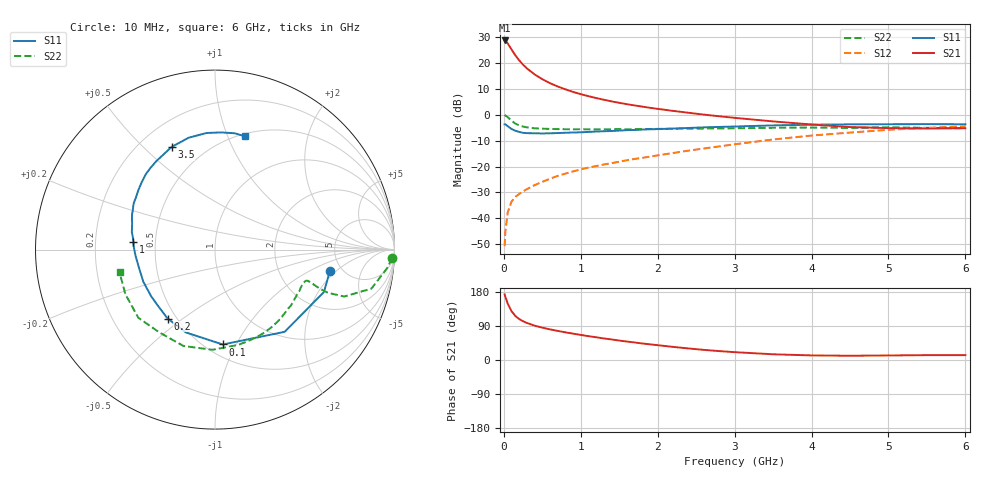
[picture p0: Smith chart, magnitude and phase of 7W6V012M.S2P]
! Infineon Technologies  Discrete & RF Semiconductors
! BFS17W
! Si NPN RF Bipolar Junction Transistor in SOT323
! VCE = 6 V  IC = 12 mA
! Common Emitter S-Parameters:  August  1999
# GHz  S  MA  R  50
!  f  S11  S21  S12  S22
! GHz  MAG  ANG  MAG  ANG  MAG  ANG  MAG  ANG
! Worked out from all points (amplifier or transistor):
!   36 points, 10 MHz to 6 GHz, reference 50 ohm
!   highest |S21| = 28.7 dB at 10 MHz (marker M1)
!   |S21| within 3 dB of that: start of sweep to 89.78 MHz
!   unconditionally stable (mu >= 1): 386.1 MHz to 2.223 GHz; 5.303 GHz to end of sweep
!   at 250 MHz: K = 0.83, MSG = 24.4 dB, |S12| = -29.6 dB
!   at 1.4 GHz: K = 1.18, MAG = 9.4 dB, |S12| = -18.7 dB
!   at 6 GHz: K = 1.04, MAG = -1.7 dB, |S12| = -4.5 dB
!   S11 on the Smith chart (normalised r, x): 10 MHz: 4.01, -1.65; 100 MHz: 0.60, -0.89; 200 MHz: 0.45, -0.44; 1 GHz: 0.37, +0.04; 3.5 GHz: 0.33, +0.61; 6 GHz: 0.53, +1.16
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0.01  0.6508 -10.5  27.08 173.4  0.0029 83.1  0.9882 -2.7
0.02  0.6515 -21.2  26.77 166.5  0.0056 84.4  0.963 -6.3
0.05  0.6004 -49.7  23.79 149.0  0.0129 69.1  0.8984 -14.0
0.1  0.5305 -85.3  18.13 128.8  0.0211 61.2  0.765 -20.0
0.15  0.4892 -109.4  13.97 116.1  0.026 56.1  0.672 -20.9
0.2  0.466 -124.5  11.18 108.1  0.0295 56.6  0.6206 -20.4
0.25  0.4459 -135.6  9.213 102.2  0.0331 56.1  0.5884 -19.6
0.3  0.4405 -144.0  7.822 97.7  0.0365 58.2  0.5702 -19.1
0.4  0.4376 -155.7  5.991 90.6  0.0437 61.0  0.5465 -18.6
0.5  0.4346 -163.5  4.842 85.4  0.0506 63.0  0.5373 -18.8
0.6  0.437 -169.3  4.055 80.8  0.058 64.9  0.5308 -19.6
0.7  0.4422 -174.3  3.505 76.8  0.0659 66.2  0.527 -20.8
0.8  0.4479 -178.7  3.083 73.0  0.0728 66.6  0.5242 -22.4
1  0.4569 174.6  2.49 66.2  0.0879 68.3  0.5241 -25.6
1.1  0.4647 170.7  2.274 62.9  0.0954 68.6  0.5221 -27.7
1.6  0.503 156.8  1.593 48.7  0.1318 70.5  0.5234 -38.9
2.2  0.5397 142.4  1.184 34.6  0.1823 72.0  0.5351 -54.3
2.8  0.5803 128.2  0.932 23.5  0.2443 70.5  0.5426 -71.1
3.5  0.6211 112.9  0.742 15.1  0.3321 65.7  0.5586 -91.6
4.5  0.6514 94.1  0.577 11.2  0.4515 53.6  0.5558 -123.8
5.5  0.6574 80.3  0.538 12.8  0.5569 40.5  0.5577 -153.5
6  0.6529 75.0  0.549 12.9  0.5986 34.0  0.5467 -166.7
